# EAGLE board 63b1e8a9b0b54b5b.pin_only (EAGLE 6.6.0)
REV: B

Size 17.78 x 19.05 mm. Coordinates in mm from the lower left corner, seen from the top.
Outline: 15.24,0 2.54,0 arc-90 0,2.54 0,16.51 arc-90 2.54,19.05 15.24,19.05 arc-90 17.78,16.51 17.78,2.54 arc-90 15.24,0
Copper layers (1*16): Top 0.035mm / dielectric 1.5mm / Bottom 0.035mm
Design rules "adafruit": minimum track width 8mil, minimum drill 15.5mil, track to track 8mil, track to pad 8mil, pad to pad 8mil, via to via 8mil, smd to smd 8mil, copper to edge 10mil, drill to drill 8mil, minimum pad ring 10mil, minimum via ring 8mil, stop-mask expansion 2mil, vias tented up to drill 20mil, thermal gap 10mil

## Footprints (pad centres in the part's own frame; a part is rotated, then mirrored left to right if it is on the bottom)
0805-NO = smd 1.3 x 1.5: 1 -0.95,0; 2 0.95,0
SOD-323 = smd 1.35 x 0.8: A 1.27,0; C -1.27,0
1X07_ROUND_70 = drill 1 pad 1.778: 1 -7.62,0; 2 -5.08,0; 3 -2.54,0; 4 0,0; 5 2.54,0; 6 5.08,0; 7 7.62,0
SOT23-WIDE = smd 1 x 1.2: 1 -0.95,-1; 2 0.95,-1; 3 0,1
_0805MP = smd 1.2 x 1.3: 1 -1.016,0; 2 1.016,0
BME280 = smd 0.7 x 0.35: 1 1.025,0.975; 2 1.025,0.325; 3 1.025,-0.325; 4 1.025,-0.975; 5 -1.025,-0.975; 6 -1.025,-0.325; 7 -1.025,0.325; 8 -1.025,0.975
SOT23-5 = smd 0.55 x 1.2: 1 -0.95,-1.3; 2 0,-1.3; 3 0.95,-1.3; 4 0.95,1.3; 5 -0.95,1.3
FIDUCIAL_1MM = smd 1 x 1: 1 0,0
MOUNTINGHOLE_2.0_PLATED = drill 2.2 pad 3: P$1 0,0

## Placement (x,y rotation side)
C1  10uF  [0805-NO]  2.29,5.84 0 top
C3  10uF  [0805-NO]  2.41,12.06 0 top
D2  1N4148  [SOD-323]  13.72,11.43 180 top
JP2  [1X07_ROUND_70]  8.89,2.54 0 top
Q3  BSS138  [SOT23-WIDE]  8.13,6.35 180 top
Q4  BSS138  [SOT23-WIDE]  14.1,6.73 180 top
R1  10K  [0805-NO]  14.1,9.53 0 top
R2  10K  [0805-NO]  8.13,9.02 0 top
R4  10K  [_0805MP]  5.21,11.05 270 top
R7  10K  [0805-NO]  5.21,6.6 90 top
R8  10K  [0805-NO]  10.92,6.6 90 top
U1  BME280  [BME280]  8.89,12.45 270 top
U2  MIC5225-3.3  [SOT23-5]  2.41,9.02 0 top
U$2  [ADAFRUIT_2.5MM]  17.53,9.02 0 bottom
U$5  FIDUCIAL""  [FIDUCIAL_1MM]  1.02,13.97 0 top
U$6  [ADAFRUIT_2.5MM]  14.86,11.94 0 top
U$7  MOUNTINGHOLE2.0  [MOUNTINGHOLE_2.0_PLATED]  2.54,16.51 0 top
U$8  MOUNTINGHOLE2.0  [MOUNTINGHOLE_2.0_PLATED]  15.24,16.51 0 top
U$15  FIDUCIAL""  [FIDUCIAL_1MM]  16.89,5.97 0 top
U$20  [PCBFEAT-REV-040]  1.4,10.03 0 bottom

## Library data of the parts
C1 C3 D2 JP2 Q3 Q4 R1 R2 R4 R7 R8 U1 U2 U$2 U$6 U$20 = microbuilder
U$5 U$7 U$8 U$15 = microbuilder; BOM: EXCLUDE

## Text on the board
tPlace: BME280 | Pressure / Temp+Humidity | VIN | GND | SDO | CS | 3Vo | SCK | SDI
bPlace: BME280 | adafruit! | Barometric Pressure / Relative Humidity / & Temperature | SPI or I2C | Vin/Vlogic: 3-5V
